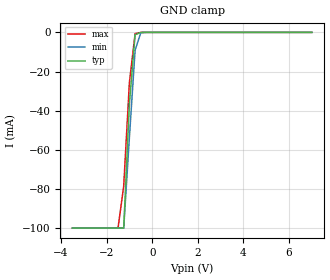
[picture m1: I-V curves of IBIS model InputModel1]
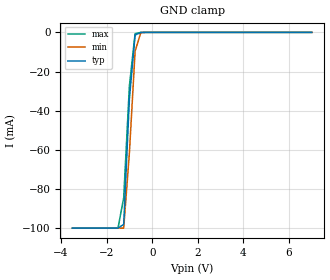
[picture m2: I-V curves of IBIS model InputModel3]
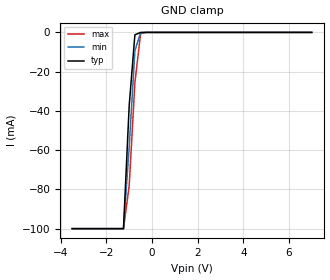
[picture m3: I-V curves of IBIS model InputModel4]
[IBIS Ver]   2.1
[File name]   da016xs3.ibs   | da= SSOP, f016xs= abbr chip name, 3= 3.3V Vcc
[File Rev]   2.00
[Date]   14-February-1996
[Source]   File generated from lab measurements at Intel Corporation
[Notes]   Rev 2.00 All data from actual measurements.
[Disclaimer] INTEL DEVELOPER'S SOFTWARE LICENSE AGREEMENT
| BY USING THIS SOFTWARE, YOU ARE AGREEING TO BE BOUND
| BY THE TERMS OFTHIS AGREEMENT.  DO NOT USE THE SOFTWARE
| UNTIL YOU HAVE CAREFULLY READAND AGREED TO THE FOLLOWING
| TERMS AND CONDITIONS.  IF YOU DO NOT AGREETO THE TERMS
| OF THIS AGREEMENT, PROMPTLY RETURN THE SOFTWARE PACKAGE
| ANDANY ACCOMPANYING ITEMS.
| IF YOU USE THIS SOFTWARE, YOU WILL BE BOUND BY THE TERMS
| OF THIS AGREEMENT
| LICENSE: Intel Corporation ("Intel") grants you the non-exclusive right
| to use the enclosed software program ("Software").  You will not use,
| copy, modify, rent, sell or transfer the Software or any portion
| thereof, except as provided in this Agreement.
| System OEM Developers may:
| 1.   Copy the Software for support, backup or archival purposes;
| 2.   Install, use, or distribute Intel owned Software in object code
|   only;
| 3.   Modify and/or use Software source code that Intel directly makes
|   available to you as an OEM Developer;
| 4.   Install, use, modify, distribute, and/or make or have made
|   derivatives ("Derivatives") of Intel owned Software under the
|   terms and conditions in this Agreement, ONLY if you are a System
|   OEM Developer and NOT an end-user.
| RESTRICTIONS:
| YOU WILL NOT:
| 1.   Copy the Software, in whole or in part, except as provided for
|   in this Agreement;
| 2.   Decompile or reverse engineer any Software provided in object
|   code format;
| 3.   Distribute any Software or Derivative code to any end-users,
|   unless approved by Intel in a prior writing.
| TRANSFER: You may transfer the Software to another OEM
| Developer if thereceiving party agrees to the terms of this
| Agreement at the sole risk of any receiving party.
| OWNERSHIP AND COPYRIGHT OF SOFTWARE:
| Title to the Software and all copies thereof remain with Intel
| or its vendors.  The Software iscopyrighted and is protected by
| United States and international copyright laws.  You will not
| remove the copyright notice from the Software.  You agree to
| prevent any unauthorized copying of the Software.
| DERIVATIVE WORK: OEM Developers that make or have made
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[Copyright]   Copyright 1996, Intel Corporation, All Rights Reserved
[Component]   DA28F016XS   | 56-lead SSOP package, 28F016XS
[Manufacturer]  Intel   | Synchronous Flash Memory
|   | operating in 3.3V Vcc range
[Package]
|Variable   typ   min   max
|The following values apply for the Copper leadframe.
R_pkg   34.81m   20.10m   46.80m
L_pkg   28.00nH   15.75nH   38.77nH
C_pkg   1.09pF   0.68pF   1.50pF
|*****************************Pin Definitions**********************************
[Pin]  signal_name   model_name   R_pin   L_pin   C_pin
  1   CE0#   InputModel1
  2   A12   InputModel1
  3   A13   InputModel1
  4   A14   InputModel3
  5   A15   InputModel1
  6   3/5#   InputModel1
  7   CE1#   InputModel1
  8   NC   InputModel2
  9   A20   InputModel3
 10   A19   InputModel3
 11   A18   InputModel1
 12   A17   InputModel1
 13   A16   InputModel1
 14   VCC   POWER
 15   GND   GND
 16   DQ6   InputOutput
 17   DQ14   InputOutput
 18   DQ7   InputOutput
 19   DQ15   InputOutput
 20   RY/BY#   OpenDrainOutput
 21   OE1#   InputModel1
 22   WE#   InputModel4
 23   WP#   InputModel1
 24   DQ13   InputOutput
 25   DQ5   InputOutput
 26   DQ12   InputOutput
 27   DQ4   InputOutput
 28   VCC   POWER
 29   GND   GND
 30   DQ11   InputOutput
 31   DQ3   InputOutput
 32   DQ10   InputOutput
 33   DQ2   InputOutput
 34   CLK   InputModel5
 35   ADV#   InputModel5
 36   BYTE#   InputModel1
 37   A0   InputModel1
 38   DQ0   InputOutput
 39   DQ8   InputOutput
 40   DQ1   InputOutput
 41   DQ9   InputOutput
 42   VCC   POWER
 43   A8   InputModel1
 44   GND   GND
 45   A7   InputModel1
 46   A6   InputModel1
 47   A5   InputModel1
 48   A4   InputModel1
 49   A3   InputModel1
 50   A2   InputModel1
 51   A1   InputModel1
 52   A9   InputModel1
 53   A10   InputModel1
 54   A11   InputModel1
 55   RP#   InputModel4
 56   VPP   POWER
|********************Input Model 2*****************************************
[Model]   InputModel2
Model_type   Input
|   for pin 8(NC)
Vinl = 0.8V
Vinh = 2.0V
| Variable   typ   min   max
C_comp   5.61p   NA   7.6p
[Voltage Range]   3.3V   3.0V   3.6V
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| Models and submodels in the file (7): InputModel1 (Input), InputModel2 (Input), InputModel3 (Input), InputModel4 (Input), InputModel5 (Input), InputOutput (I/O), OpenDrainOutput (Open_drain)
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|*********************Inoput Model 1***************************************
[Model]   InputModel1
Model_type   Input
|   for pin1(3/5#), CE1#, CE0#, OE#, WP#, BYTE#, A[18:15], A[13:0]
Vinl = 0.8V
Vinh = 2.0V
| Variable   typ   min   max
C_comp   5.61p   NA   7.6p
[Voltage Range]   3.3V   3.0V   3.6V
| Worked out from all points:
|   GND clamp passes 1 mA (typ) near -0.71 V on its own axis
[GND_clamp]
|Voltage I(typ)   I(min)   I(max)
-3.5V     -99.93mA   -99.94mA   -99.95mA
-1.5V     -99.93mA   -99.94mA   -99.95mA
-1.25V    -99.93mA   -99.94mA   -78.52mA
-1V       -36.25mA   -53.59mA   -25.61mA
-750mV    -1.199mA   -9.118mA   -666.9uA
-500mV    -23uA      -169.3uA   -33.07uA
7V        0A         0A         0A
[POWER_clamp]
| Input buffer circuits of this product do not intrinsically
| require a [POWER_clamp] definition.  This zero current
| [POWER_clamp] is provided for compatibility with some ibis
| parsers.
|   Voltage  I(typ)   I(min)   I(max)
-3.3V     0A         0A         0A
-3V       0A         0A         0A
6.3V      0A         0A         0A
6.6V      0A         0A         0A
|*******************Input Model 3**************************************
[Model]   InputModel3
Model_type   Input
|   for A[20], A[19], A[14]
Vinl = 0.8V
Vinh = 2.0V
| Variable   typ   min   max
C_comp   5.61p   NA   7.6p
[Voltage Range]   3.3V   3.0V   3.6V
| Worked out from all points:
|   GND clamp passes 1 mA (typ) near -0.68 V on its own axis
[GND_clamp]
|Voltage I(typ)   I(min)   I(max)
-3.5V     -99.93mA   -99.94mA   -99.95mA
-1.5V     -99.93mA   -99.94mA   -99.95mA
-1.25V    -98.01mA   -99.94mA   -84.37mA
-1V       -33.88mA   -61.45mA   -27.19mA
-750mV    -1.338mA   -9.608mA   -639.5uA
-500mV    -54.63uA   -152.9uA   0A
7V        0A         0A         0A
[POWER_clamp]
| Input buffer circuits of this product do not intrinsically
| require a [POWER_clamp] definition.  This zero current
| [POWER_clamp] is provided for compatibility with some ibis
| parsers.
|   Voltage  I(typ)   I(min)   I(max)
-3.3V     0A         0A         0A
-3V       0A         0A         0A
6.3V      0A         0A         0A
6.6V      0A         0A         0A
|*********************Input Model 4*************************************
[Model]   InputModel4
Model_type   Input
|   for RP#, WE#
Vinl = 0.8V
Vinh = 2.0V
| Variable   typ   min   max
C_comp   5.61p   NA   7.6p
[Voltage Range]   3.3V   3.0V   3.6V
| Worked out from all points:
|   GND clamp passes 1 mA (typ) near -0.70 V on its own axis
[GND_clamp]
|Voltage I(typ)   I(min)   I(max)
-3.5V     -99.94mA   -99.94mA   -99.95mA
-1.25V    -99.94mA   -99.94mA   -99.95mA
-1V       -37.36mA   -58.41mA   -78.12mA
-750mV    -1.233mA   -9.326mA   -25.63mA
-500mV    -23.22uA   -151.2uA   -617uA
-250mV    0A         0A         0A
7V        0A         0A         0A
[POWER_clamp]
| Input buffer circuits of this product do not intrinsically
| require a [POWER_clamp] definition.  This zero current
| [POWER_clamp] is provided for compatibility with some ibis
| parsers.
|   Voltage  I(typ)   I(min)   I(max)
-3.3V     0A         0A         0A
-3V       0A         0A         0A
6.3V      0A         0A         0A
6.6V      0A         0A         0A
